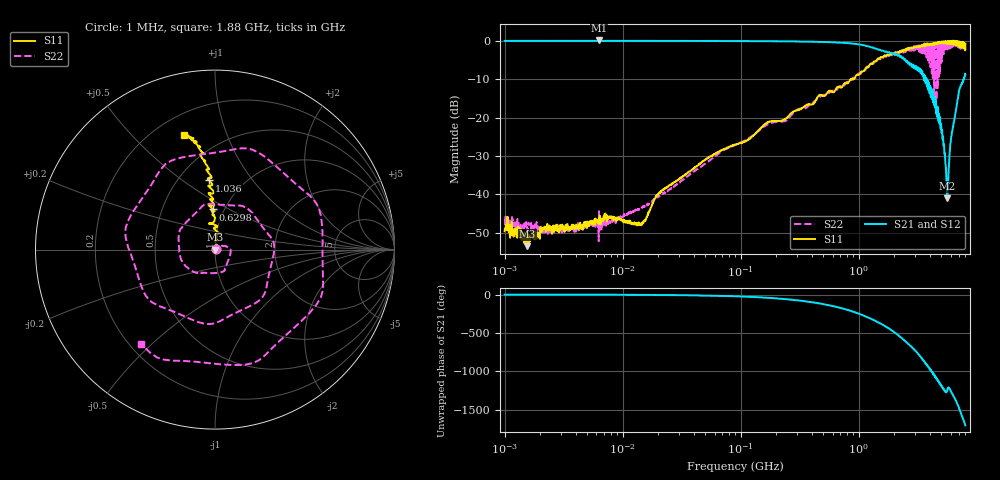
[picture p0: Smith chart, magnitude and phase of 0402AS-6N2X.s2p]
!s-Parameter Generated by FASTRON Sdn. Bhd.
!FASTRON P/N : 0402AS-6N2X
!Keysight Technologies: E5071C_MY46733604_B.14.02
!Date: Mon Dec 01 10:25:09 2025
!Version  :Rev00  Mon Dec 01 10:25:09 2025
!Data & Calibration Information:
!Freq  S11:SOLT2(ON)  S21:SOLT2(ON)  S12:SOLT2(ON)  S22:SOLT2(ON)
!PortZ  Port1:50+j0  Port2:50+j0
!When reading reference impedance value at option line is always used.
! Remarks : This data is being provided solely for informational purposes.
# Hz S dB R 50
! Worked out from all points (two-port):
!   1601 points, 1 MHz to 8 GHz, reference 50 ohm
!   highest |S21| = 0.07 dB at 6.301 MHz (marker M1); lowest = -41.0 dB at 5.612 GHz (marker M2)
!   |S21| within 3 dB of the highest: start of sweep to 1.729 GHz
!   lowest |S11| = -53.5 dB at 1.559 MHz (marker M3), VSWR 1.00, Z = 50.2 + j0.0506 ohm
!   |S11| at or under -10 dB: start of sweep to 856.3 MHz; 878.7 MHz to 901.2 MHz (22.46 MHz wide, 2.52 % of centre)
!   |S22| runs from -52.2 to -0.3 dB; largest |S21 - S12| = 0.016
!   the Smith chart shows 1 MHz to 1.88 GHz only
!   S11 on the Smith chart (normalised r, x): 1 MHz: 1.01, +0.00; 629.8 MHz: 0.89, +0.42; 1.036 GHz: 0.70, +0.64; 1.88 GHz: 0.32, +0.72
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1000000  -49.60 19.8  -0.05 -0.2  -0.03 -0.2  -46.90 13.5
1559194  -53.50 13.8  -0.04 -0.4  -0.04 -0.4  -48.50 -0.1
4479405  -48.40 31.8  -0.05 -1.1  -0.03 -1.2  -48.70 37.1
6301378  -46.10 51.1  0.07 -1.5  0.06 -1.1  -44.40 34.1
2.00676e7  -39.90 47.8  -0.05 -5.1  -0.05 -5.1  -40.50 64.3
8.994653e7  -27.00 88.8  -0.08 -22.7  -0.08 -22.7  -27.10 28.9
4.006501e8  -16.60 98.9  -0.25 -99.8  -0.24 -99.8  -16.30 -122.0
6.29833e8  -13.00 92.7  -0.42 -157.0  -0.41 -157.0  -13.10 134.0
1.035959e9  -8.26 94.7  -1.01 102.0  -1.01 102.0  -8.64 -71.4
1.442356e9  -4.70 99.3  -2.25 1.9  -2.24 1.8  -5.01 81.1
1.7949e9  -3.77 104.0  -2.95 -80.7  -2.95 -80.8  -3.88 -87.4
1.88012e9  -3.60 105.0  -3.17 -101.0  -3.18 -101.0  -3.51 -128.0
2.157084e9  -3.05 109.0  -3.89 -168.0  -3.89 -168.0  -2.80 95.8
2.516241e9  -2.10 116.0  -5.41 103.0  -5.39 103.0  -2.37 -93.9
2.721653e9  -1.83 118.0  -6.41 56.0  -6.38 55.9  -1.81 170.0
2.89772e9  -1.66 123.0  -6.79 13.9  -6.76 13.8  -2.20 78.9
3.244011e9  -1.63 128.0  -7.21 -64.5  -7.18 -64.8  -1.89 -75.8
3.588581e9  -0.91 141.0  -10.40 -153.0  -10.30 -153.0  -1.62 82.8
3.95342e9  -0.89 141.0  -12.30 116.0  -12.30 115.0  -5.99 -99.4
4.324643e9  -1.02 146.0  -14.50 28.8  -14.60 28.3  -4.05 126.0
5.612268e9  -0.58 -176.0  -41.00 -170.0  -41.10 -170.0  -1.13 -130.0
8e9  -0.79 -105.0  -8.77 98.0  -8.80 97.7  -2.35 137.0
